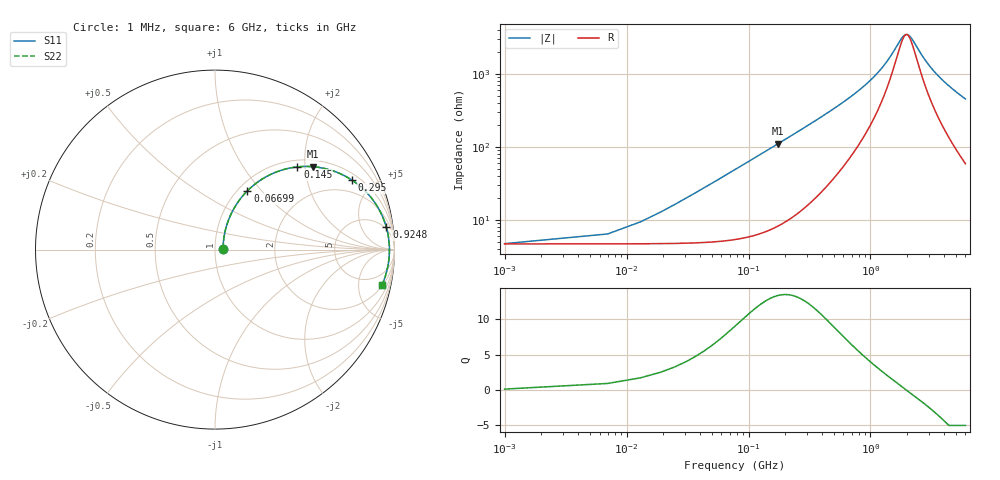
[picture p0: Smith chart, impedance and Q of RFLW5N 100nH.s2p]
!Vishay Electro-Films
!RFLW5N1000A - 100 nH Spiral Inductor on Quartz
!Measured in series configuration
!May 2011
# GHz S MA R 50
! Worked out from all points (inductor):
!   1001 points, 1 MHz to 6 GHz, reference 50 ohm
!   read as one part in series: L = 99.7 nH near 31 MHz
!   highest Q = 13.3 at 175 MHz (marker M1), where L = 100 nH
!   self-resonance near 1.974 GHz
!   S11 on the Smith chart (normalised r, x): 1 MHz: 1.09, +0.01; 66.99 MHz: 1.10, +0.84; 145 MHz: 1.14, +1.83; 295 MHz: 1.30, +3.77; 924.8 MHz: 4, +14; 6 GHz: 2.18, -9.00
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0.001  0.04523 7.3  0.9551 -0.3  0.9551 -0.3  0.04523 7.3
0.018997  0.1215 61.8  0.9487 -6.5  0.9487 -6.5  0.1215 61.8
0.042993  0.2529 65.3  0.9233 -14.4  0.9233 -14.4  0.2529 65.3
0.066989  0.3737 61.2  0.8827 -21.8  0.8827 -21.8  0.3737 61.2
0.102983  0.5234 53.4  0.8058 -31.4  0.8058 -31.4  0.5234 53.4
0.144976  0.6505 45.1  0.7105 -40.4  0.7105 -40.4  0.6505 45.1
0.174971  0.716 40.2  0.6468 -45.6  0.6468 -45.6  0.716 40.2
0.228962  0.797 33.1  0.5475 -52.6  0.5475 -52.6  0.797 33.1
0.294951  0.8562 26.8  0.4528 -58.6  0.4528 -58.6  0.8562 26.8
0.390935  0.9028 20.7  0.3545 -64.0  0.3545 -64.0  0.9028 20.7
0.510915  0.9318 15.7  0.2725 -67.8  0.2725 -67.8  0.9318 15.7
0.924846  0.9628 7.4  0.1325 -70.0  0.1325 -70.0  0.9628 7.4
1.00283  0.9648 6.5  0.1172 -69.3  0.1172 -69.3  0.9648 6.5
1.76471  0.9717 1.0  0.03319 -31.0  0.03319 -31.0  0.9717 1.0
1.89069  0.9719 0.4  0.02889 -13.2  0.02889 -13.2  0.9719 0.4
2.00467  0.9719 -0.1  0.02816 4.8  0.02816 4.8  0.9719 -0.1
2.15464  0.9719 -0.8  0.0312 25.3  0.0312 25.3  0.9719 -0.8
2.66456  0.971 -2.7  0.05523 56.9  0.05523 56.9  0.971 -2.7
3.0005  0.9699 -3.9  0.07293 63.7  0.07293 63.7  0.9699 -3.9
4.00233  0.9652 -6.9  0.1225 70.1  0.1225 70.1  0.9652 -6.9
5.00417  0.9588 -9.5  0.1677 71.1  0.1677 71.1  0.9588 -9.5
6  0.951 -12.0  0.2096 70.5  0.2096 70.5  0.951 -12.0
